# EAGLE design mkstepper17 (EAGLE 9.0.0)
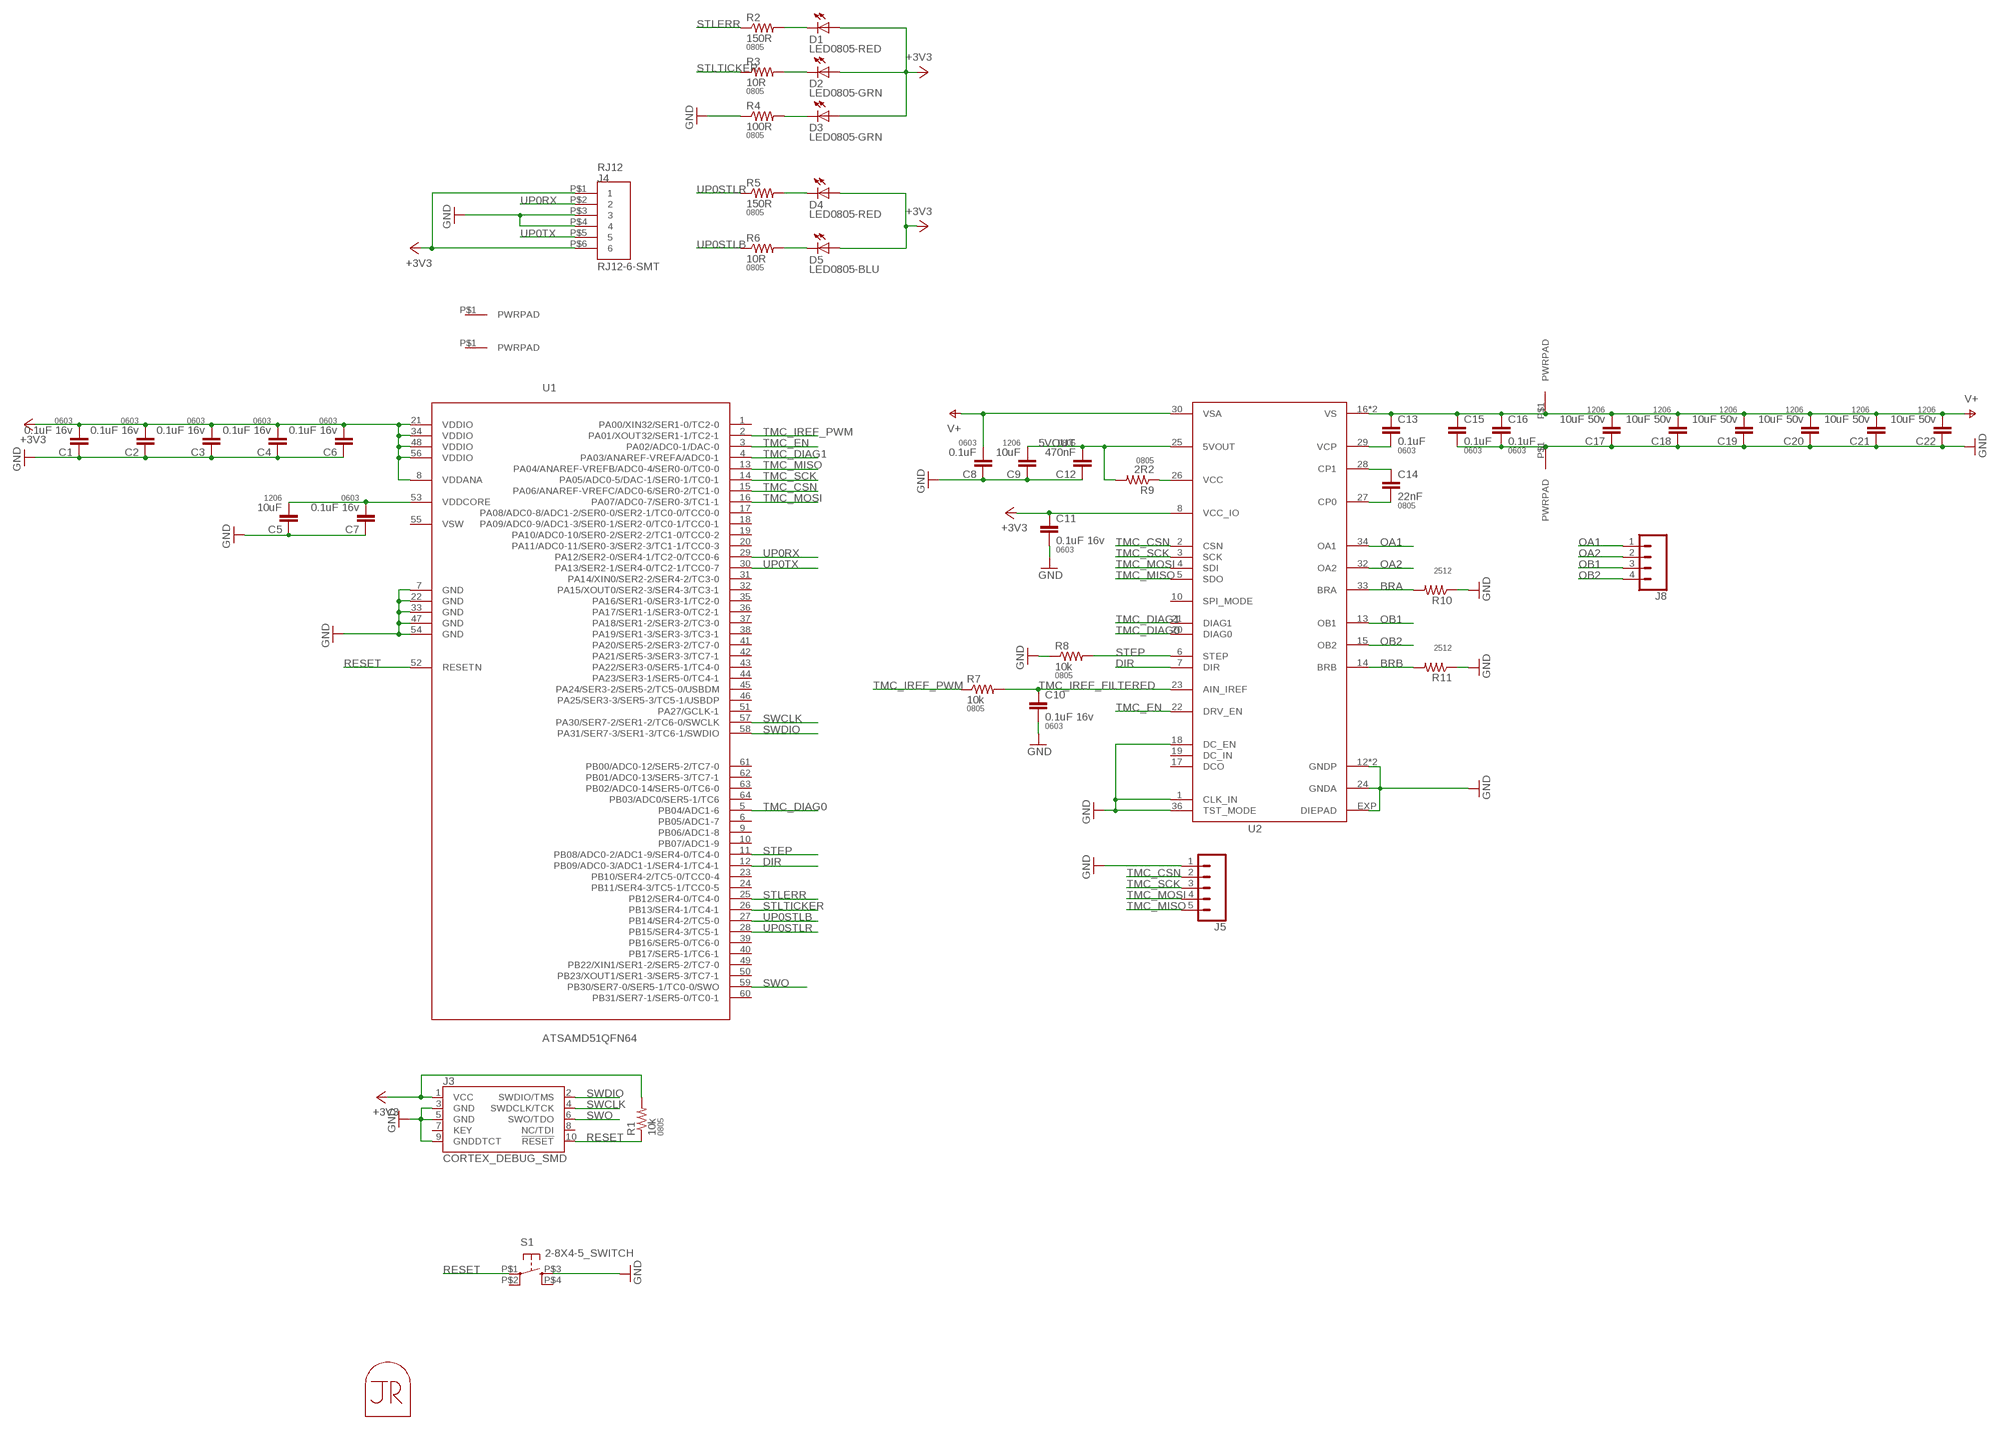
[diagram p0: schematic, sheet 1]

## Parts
C1  0.1uF 16v  CAP0603-CAP  [0603-CAP]
C2  0.1uF 16v  CAP0603-CAP  [0603-CAP]
C3  0.1uF 16v  CAP0603-CAP  [0603-CAP]
C4  0.1uF 16v  CAP0603-CAP  [0603-CAP]
C5  10uF  CAP1206  [1206]
C6  0.1uF 16v  CAP0603-CAP  [0603-CAP]
C7  0.1uF 16v  CAP0603-CAP  [0603-CAP]
C8  0.1uF  CAP0603-CAP  [0603-CAP]
C9  10uF  CAP1206  [1206]
C10  0.1uF 16v  CAP0603-CAP  [0603-CAP]
C11  0.1uF 16v  CAP0603-CAP  [0603-CAP]
C12  470nF  CAP0805  [0805]
C13  0.1uF  CAP0603-CAP  [0603-CAP]
C14  22nF  CAP0805  [0805]
C15  0.1uF  CAP0603-CAP  [0603-CAP]
C16  0.1uF  CAP0603-CAP  [0603-CAP]
C17  10uF 50v  CAP1206  [1206]
C18  10uF 50v  CAP1206  [1206]
C19  10uF 50v  CAP1206  [1206]
C20  10uF 50v  CAP1206  [1206]
C21  10uF 50v  CAP1206  [1206]
C22  10uF 50v  CAP1206  [1206]
D1  LED0805-RED  LED0805  [LED0805]
D2  LED0805-GRN  LED0805  [LED0805]
D3  LED0805-GRN  LED0805  [LED0805]
D4  LED0805-RED  LED0805  [LED0805]
D5  LED0805-BLU  LED0805  [LED0805]
J1  PWRPADM3  [PWRPAD_3-25MM]
J2  PWRPADM3  [PWRPAD_3-25MM]
J3  CORTEX_DEBUG_SMD  [SAMTECH_FTSH-105-01]
J4  RJ12-6-SMT  [RJ12-6-SMT]
J5  CONN_05NO_SILK  [1X05_NO_SILK]
J6  PWRPAD  [PWRPAD_M3-PEM-MOUNT]
J7  PWRPAD  [PWRPAD_M3-PEM-MOUNT]
J8  CONN_04LONGPADS  [1X04_LONGPADS]
MP1  JRTOMBSTONE  [JRTOMBSTONE]
R1  10k  RESISTOR0805-RES  [0805]
R2  150R  RESISTOR0805-RES  [0805]
R3  10R  RESISTOR0805-RES  [0805]
R4  100R  RESISTOR0805-RES  [0805]
R5  150R  RESISTOR0805-RES  [0805]
R6  10R  RESISTOR0805-RES  [0805]
R7  10k  RESISTOR0805-RES  [0805]
R8  10k  RESISTOR0805-RES  [0805]
R9  2R2  RESISTOR0805-RES  [0805]
R10  RESISTOR2512  [R2512]
R11  RESISTOR2512  [R2512]
S1  2-8X4-5_SWITCH  [TACT-SWITCH-KMR6]
U1  ATSAMD51QFN64  [QFN-64-9X9MM]
U2  TMC2130  [QFN36-5X6]

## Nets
5VOUT: C9.2 C12.2 R9.2 U2.25(5VOUT)
+3V3: C1.2 C2.2 C3.2 C4.2 C6.2 C11.1 D1.1(A) D2.1(A) D3.1(A) D4.1(A) D5.1(A) J3.1(VCC) J4.P$1 J4.P$6 R1.2 U1.8(VDDANA) U1.21(VDDIO) U1.34(VDDIO) U1.48(VDDIO) U1.56(VDDIO) U2.8(VCC_IO)
BRA: R10.2 U2.33(BRA)
BRB: R11.2 U2.14(BRB)
DIR: U1.12(PB09/ADC0-3/ADC1-1/SER4-1/TC4-1) U2.7(DIR)
GND: C1.1 C2.1 C3.1 C4.1 C5.1 C6.1 C7.1 C8.1 C9.1 C10.2 C11.2 C12.1 C15.2 C16.2 C17.1 C18.1 C19.1 C20.1 C21.1 C22.1 J3.3(GND) J3.5(GND) J3.9(GNDDTCT) J4.P$3 J4.P$4 J5.1 J7.P$1(PWRPAD) R4.1 R8.1 R10.1 R11.1 S1.P$3(S) U1.7(GND) U1.22(GND) U1.33(GND) U1.47(GND) U1.54(GND) U2.1(CLK_IN) U2.12(GNDP) U2.18(DC_EN) U2.24(GNDA) U2.35(GNDP) U2.36(TST_MODE) U2.EXP(DIEPAD)
N$1: D3.2(C) R4.2
N$5: D2.2(C) R3.2
N$6: D1.2(C) R2.2
N$7: C5.2 C7.2 U1.53(VDDCORE)
N$10: D4.2(C) R5.2
N$11: D5.2(C) R6.2
N$12: C14.2 U2.27(CP0)
N$13: R9.1 U2.26(VCC)
N$14: C14.1 U2.28(CP1)
N$15: C13.2 U2.29(VCP)
OA1: J8.1 U2.34(OA1)
OA2: J8.2 U2.32(OA2)
OB1: J8.3 U2.13(OB1)
OB2: J8.4 U2.15(OB2)
RESET: J3.10(!RESET) R1.1 S1.P$1(P) U1.52(RESETN)
STEP: R8.2 U1.11(PB08/ADC0-2/ADC1-9/SER4-0/TC4-0) U2.6(STEP)
STLERR: R2.1 U1.25(PB12/SER4-0/TC4-0)
STLTICKER: R3.1 U1.26(PB13/SER4-1/TC4-1)
SWCLK: J3.4(SWDCLK/TCK) U1.57(PA30/SER7-2/SER1-2/TC6-0/SWCLK)
SWDIO: J3.2(SWDIO/TMS) U1.58(PA31/SER7-3/SER1-3/TC6-1/SWDIO)
SWO: J3.6(SWO/TDO) U1.59(PB30/SER7-0/SER5-1/TC0-0/SWO)
TMC_CSN: J5.2 U1.15(PA06/ANAREF-VREFC/ADC0-6/SER0-2/TC1-0) U2.2(CSN)
TMC_DIAG0: U1.5(PB04/ADC1-6) U2.20(DIAG0)
TMC_DIAG1: U1.4(PA03/ANAREF-VREFA/ADC0-1) U2.21(DIAG1)
TMC_EN: U1.3(PA02/ADC0-1/DAC-0) U2.22(DRV_EN)
TMC_IREF_FILTERED: C10.1 R7.2 U2.23(AIN_IREF)
TMC_IREF_PWM: R7.1 U1.2(PA01/XOUT32/SER1-1/TC2-1)
TMC_MISO: J5.5 U1.13(PA04/ANAREF-VREFB/ADC0-4/SER0-0/TC0-0) U2.5(SDO)
TMC_MOSI: J5.4 U1.16(PA07/ADC0-7/SER0-3/TC1-1) U2.4(SDI)
TMC_SCK: J5.3 U1.14(PA05/ADC0-5/DAC-1/SER0-1/TC0-1) U2.3(SCK)
UP0RX: J4.P$2 U1.29(PA12/SER2-0/SER4-1/TC2-0/TCC0-6)
UP0STLB: R6.1 U1.27(PB14/SER4-2/TC5-0)
UP0STLR: R5.1 U1.28(PB15/SER4-3/TC5-1)
UP0TX: J4.P$5 U1.30(PA13/SER2-1/SER4-0/TC2-1/TCC0-7)
V+: C8.2 C13.1 C15.1 C16.1 C17.2 C18.2 C19.2 C20.2 C21.2 C22.2 J6.P$1(PWRPAD) U2.16(VS) U2.30(VSA) U2.31(VS)
Unconnected: J1.P$1(PWRPAD) J2.P$1(PWRPAD) J3.7(KEY) J3.8(NC/TDI) S1.P$2(P1) S1.P$4(S1) U1.1(PA00/XIN32/SER1-0/TC2-0) U1.6(PB05/ADC1-7) U1.9(PB06/ADC1-8) U1.10(PB07/ADC1-9) U1.17(PA08/ADC0-8/ADC1-2/SER0-0/SER2-1/TC0-0/TCC0-0) U1.18(PA09/ADC0-9/ADC1-3/SER0-1/SER2-0/TC0-1/TCC0-1) U1.19(PA10/ADC0-10/SER0-2/SER2-2/TC1-0/TCC0-2) U1.20(PA11/ADC0-11/SER0-3/SER2-3/TC1-1/TCC0-3) U1.23(PB10/SER4-2/TC5-0/TCC0-4) U1.24(PB11/SER4-3/TC5-1/TCC0-5) U1.31(PA14/XIN0/SER2-2/SER4-2/TC3-0) U1.32(PA15/XOUT0/SER2-3/SER4-3/TC3-1) U1.35(PA16/SER1-0/SER3-1/TC2-0) U1.36(PA17/SER1-1/SER3-0/TC2-1) U1.37(PA18/SER1-2/SER3-2/TC3-0) U1.38(PA19/SER1-3/SER3-3/TC3-1) U1.39(PB16/SER5-0/TC6-0) U1.40(PB17/SER5-1/TC6-1) U1.41(PA20/SER5-2/SER3-2/TC7-0) U1.42(PA21/SER5-3/SER3-3/TC7-1) U1.43(PA22/SER3-0/SER5-1/TC4-0) U1.44(PA23/SER3-1/SER5-0/TC4-1) U1.45(PA24/SER3-2/SER5-2/TC5-0/USBDM) U1.46(PA25/SER3-3/SER5-3/TC5-1/USBDP) U1.49(PB22/XIN1/SER1-2/SER5-2/TC7-0) U1.50(PB23/XOUT1/SER1-3/SER5-3/TC7-1) U1.51(PA27/GCLK-1) U1.55(VSW) U1.60(PB31/SER7-1/SER5-0/TC0-1) U1.61(PB00/ADC0-12/SER5-2/TC7-0) U1.62(PB01/ADC0-13/SER5-3/TC7-1) U1.63(PB02/ADC0-14/SER5-0/TC6-0) U1.64(PB03/ADC0/SER5-1/TC6) U2.10(SPI_MODE) U2.17(DCO) U2.19(DC_IN)

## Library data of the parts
C1-C4 C6-C8 C10 C11 C13 C15 C16 = borkedlabs-passives:CAP: Capacitor; PACKAGE: 0603
C5 C9 C17-C22 = borkedlabs-passives:CAP: Capacitor; PACKAGE: 1206
C12 C14 = borkedlabs-passives:CAP: Capacitor; PACKAGE: 0805
D1-D5 = lights:LED: LED
J1 J2 J6 J7 = power:PWRPAD
J3 = SparkFun-Connectors:CORTEX_DEBUG: Cortex Debug Connector - 10 pin Supports JTAG debug, Serial Wire debug, and Serial Wire Viewer. PTH and SMD connector options available. General Connector Information Products: PTH Connector -via Digi-Key SparkFun PSoc SparkFun T
J4 = connector:RJ12-6-SMT
J5 = SparkFun-Connectors:CONN_05: Multi connection point. Often used as Generic Header-pin footprint for 0.1 inch spaced/style header connections On any of the 0.1 inch spaced packages, you can populate with these: Break Away Headers - Straight (PRT-00116) Break Away Male Headers - Right Angle (PRT-00553) Female Headers (PRT-00115)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
J8 = SparkFun-Connectors:CONN_04: Multi connection point. Often used as Generic Header-pin footprint for 0.1 inch spaced/style header connections On any of the 0.1 inch spaced packages, you can populate with these: Break Away Headers - Straight (PRT-00116) Break Away Male Headers - Right Angle (PRT-00553) Female Headers (PRT-00115)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; PROD_ID: CONN-09696
MP1 = connector:JRTOMBSTONE
R1-R9 = borkedlabs-passives:RESISTOR: Resistor; PACKAGE: 0805
R10 R11 = borkedlabs-passives:RESISTOR: Resistor; PACKAGE: 2512
S1 = fab:2-8X4-5_SWITCH
U1 = atsam:ATSAMD51
U2 = power:TMC2130

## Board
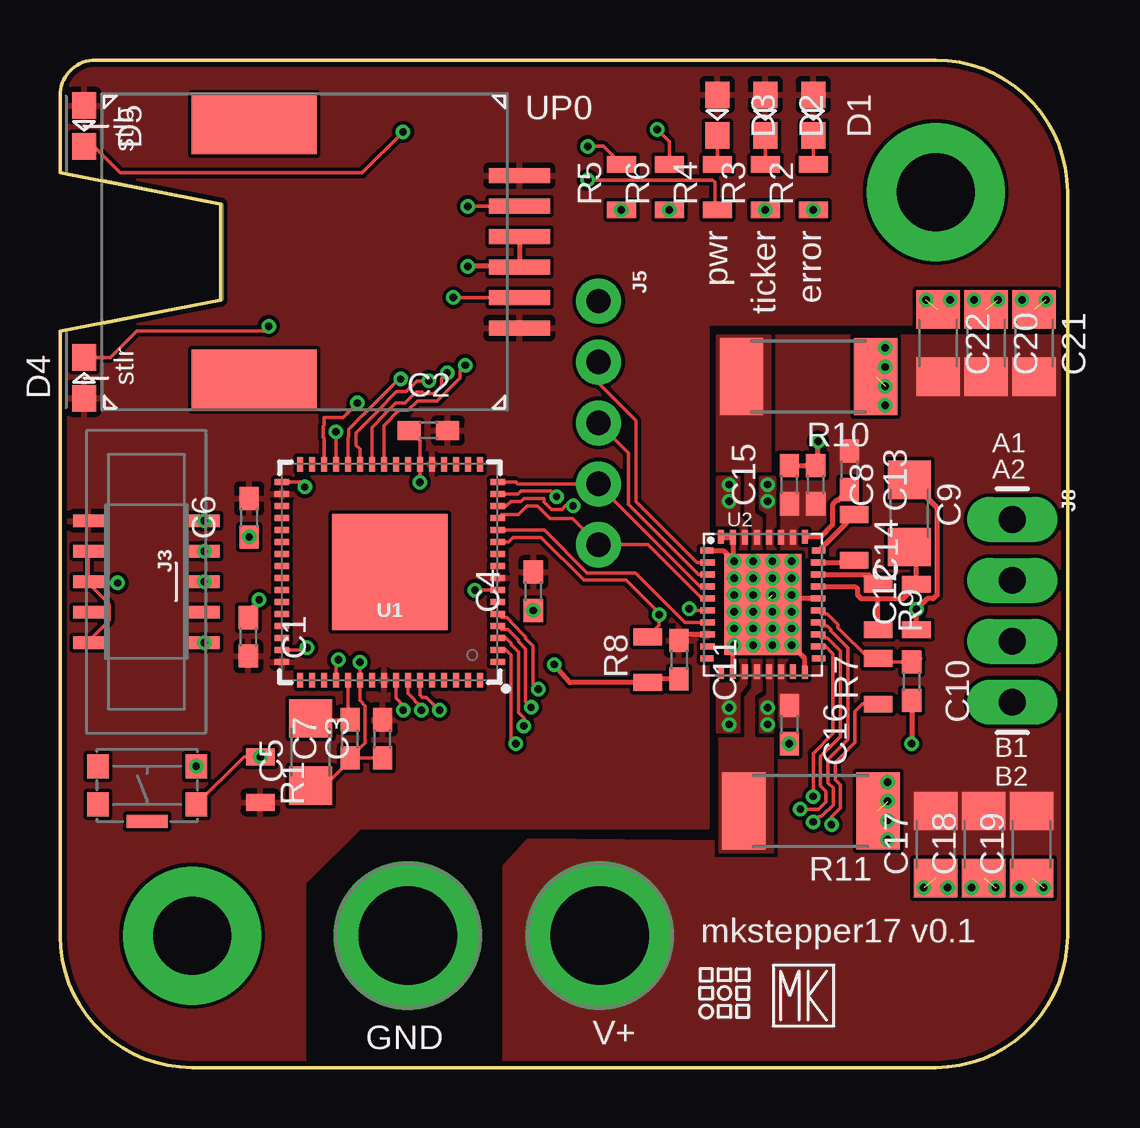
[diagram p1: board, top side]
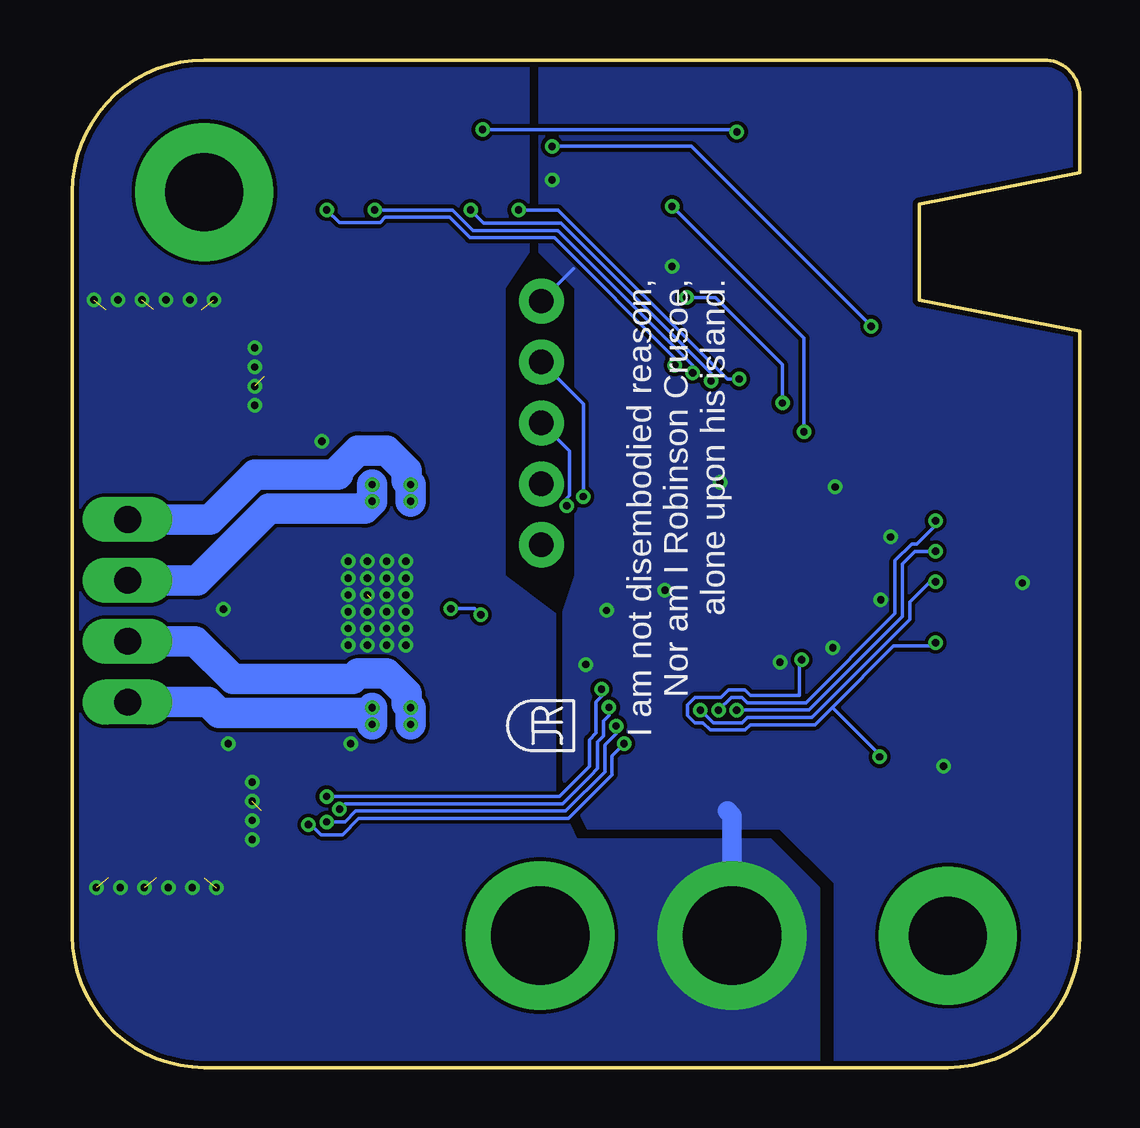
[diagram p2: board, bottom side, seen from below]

Size 42 x 42 mm. Coordinates in mm from the lower left corner, seen from the top.
Outline: 5.5,0 36.5,0 arc90 42,5.5 42,36.5 arc90 36.5,42 1.5,42 arc90 0,40.5 0,37.3 6.7,36 6.7,32 0,30.7 0,5.5 arc90 5.5,0
Copper layers (1*16): Top 0.035mm / dielectric 1.5mm / Bottom 0.035mm
Design rules "default *": minimum track width 6mil, minimum drill 0.3mm, track to track 6mil, track to pad 6mil, pad to pad 6mil, via to via 6mil, smd to smd 6mil, copper to edge 8mil, drill to drill 8mil, minimum pad ring 6mil, minimum via ring 6mil, stop-mask expansion 4mil, vias tented up to drill 27mil, thermal gap 9mil

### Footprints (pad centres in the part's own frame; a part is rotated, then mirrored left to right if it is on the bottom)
0603-CAP = smd 0.96 x 0.8: 1 -0.8,0; 2 0.8,0
1206 = smd 1.6 x 1.8: 1 -1.4,0; 2 1.4,0
0805 = smd 0.7 x 1.2: 1 -0.95,0; 2 0.95,0
LED0805 = smd 1.1 x 1: 1 -0.85,0; 2 0.85,0
PWRPAD_3-25MM = drill 3.25 pad 5.75: P$1 0,0
SAMTECH_FTSH-105-01 = smd 0.508 x 1.27: 1 -2.54,-2.413; 2 -2.54,2.413; 3 -1.27,-2.413; 4 -1.27,2.413; 5 0,-2.413; 6 0,2.413; 7 1.27,-2.413; 8 1.27,2.413; 9 2.54,-2.413; 10 2.54,2.413
RJ12-6-SMT = smd 0.635 x 2.54: P$1 -3.175,17.399; P$2 -1.905,17.399; P$3 -0.635,17.399; P$4 0.635,17.399; P$5 1.905,17.399; P$6 3.175,17.399 | smd 2.54 x 5.207: P$7 -5.334,6.35; P$8 5.334,6.35
1X05_NO_SILK = drill 1.016 pad 1.88: 1 0,0; 2 2.54,0; 3 5.08,0; 4 7.62,0; 5 10.16,0
PWRPAD_M3-PEM-MOUNT = drill 4.1 pad 6.2: P$1 0,0
1X04_LONGPADS = drill 1.118 pad 1.88 long: 1 0,0; 2 2.54,0; 3 5.08,0; 4 7.62,0
R2512 = smd 1.8 x 3.2: 1 -2.8,0; 2 2.8,0
TACT-SWITCH-KMR6 = smd 0.9 x 1: P$1 -2.05,0.8; P$2 2.05,0.8; P$3 -2.05,-0.8; P$4 2.05,-0.8 | smd 1.7 x 0.55: P$5 0,1.5
QFN-64-9X9MM = smd 0.6 x 0.25: 1 -4.5,3.75; 2 -4.5,3.25; 3 -4.5,2.75; 4 -4.5,2.25; 5 -4.5,1.75; 6 -4.5,1.25; 7 -4.5,0.75; 8 -4.5,0.25; 9 -4.5,-0.25; 10 -4.5,-0.75; 11 -4.5,-1.25; 12 -4.5,-1.75; 13 -4.5,-2.25; 14 -4.5,-2.75; 15 -4.5,-3.25; 16 -4.5,-3.75; 33 4.5,-3.75; 34 4.5,-3.25; 35 4.5,-2.75; 36 4.5,-2.25; 37 4.5,-1.75; 38 4.5,-1.25; 39 4.5,-0.75; 40 4.5,-0.25; 41 4.5,0.25; 42 4.5,0.75; 43 4.5,1.25; 44 4.5,1.75; 45 4.5,2.25; 46 4.5,2.75; 47 4.5,3.25; 48 4.5,3.75 | smd 0.25 x 0.6: 17 -3.75,-4.5; 18 -3.25,-4.5; 19 -2.75,-4.5; 20 -2.25,-4.5; 21 -1.75,-4.5; 22 -1.25,-4.5; 23 -0.75,-4.5; 24 -0.25,-4.5; 25 0.25,-4.5; 26 0.75,-4.5; 27 1.25,-4.5; 28 1.75,-4.5; 29 2.25,-4.5; 30 2.75,-4.5; 31 3.25,-4.5; 32 3.75,-4.5; 49 3.75,4.5; 50 3.25,4.5; 51 2.75,4.5; 52 2.25,4.5; 53 1.75,4.5; 54 1.25,4.5; 55 0.75,4.5; 56 0.25,4.5; 57 -0.25,4.5; 58 -0.75,4.5; 59 -1.25,4.5; 60 -1.75,4.5; 61 -2.25,4.5; 62 -2.75,4.5; 63 -3.25,4.5; 64 -3.75,4.5 | smd 4.826 x 4.826: P$1 0,0
QFN36-5X6 = smd 0.55 x 0.25: 1 -2.325,1.75; 10 -2.325,-2.75; 19 2.325,-2.75; 28 2.325,1.75 | smd 0.6 x 0.25: 2 -2.3,1.25; 3 -2.3,0.75; 4 -2.3,0.25; 5 -2.3,-0.25; 6 -2.3,-0.75; 7 -2.3,-1.25; 8 -2.3,-1.75; 9 -2.3,-2.25; 20 2.3,-2.25; 21 2.3,-1.75; 22 2.3,-1.25; 23 2.3,-0.75; 24 2.3,-0.25; 25 2.3,0.25; 26 2.3,0.75; 27 2.3,1.25 | smd 0.25 x 0.55: 11 -1.75,-3.325; 18 1.75,-3.325; 29 1.75,2.325; 36 -1.75,2.325 | smd 0.25 x 0.6: 12 -1.25,-3.3; 13 -0.75,-3.3; 14 -0.25,-3.3; 15 0.25,-3.3; 16 0.75,-3.3; 17 1.25,-3.3; 30 1.25,2.3; 31 0.75,2.3; 32 0.25,2.3; 33 -0.25,2.3; 34 -0.75,2.3; 35 -1.25,2.3 | smd 3.2 x 4.2: EXP 0,-0.5

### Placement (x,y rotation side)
C1  7.85,17.95 270 top
C2  15.36,26.55 0 top
C3  13.45,13.7 90 top
C4  19.73,19.85 90 top
C5  10.45,13.15 90 top
C6  7.89,22.92 90 top
C7  12.1,13.7 90 top
C8  31.5,24.3 270 top
C9  35.4,23.1 270 top
C10  35.5,16.1 270 top
C11  25.8,17 270 top
C12  35.7,19.2 90 top
C13  32.9,24.9 270 top
C14  33.1,22.1 270 top
C15  30.4,24.3 90 top
C16  30.4,14.3 270 top
C17  36.5,9.3 90 top
C18  38.5,9.3 90 top
C19  40.5,9.3 90 top
C20  38.6,30.2 270 top
C21  40.6,30.2 270 top
C22  36.6,30.2 270 top
D1  31.4,39.7 270 top
D2  29.4,39.7 270 top
D3  27.4,39.7 270 top
D4  1,28.75 90 top
D5  1,39.25 270 top
J1  36.5,36.5 0 top
J2  5.5,5.5 0 top
J3  3.6,20.25 270 top
J4  1.75,34 270 top
J5  22.45,31.95 270 top
J6  22.5,5.5 0 top
J7  14.5,5.5 0 top
J8  39.7,22.85 270 top
MP1  22.1,14.3 90 bottom
R1  8.35,12 270 top
R2  31.4,36.7 90 top
R3  29.4,36.7 90 top
R4  27.4,36.7 90 top
R5  23.4,36.7 90 top
R6  25.4,36.7 90 top
R7  34.1,16.1 90 top
R8  24.5,17 90 top
R9  34.1,19.2 270 top
R10  31.2,28.8 180 top
R11  31.3,10.7 180 top
S1  3.63,11.76 180 top
U1  13.75,20.65 180 top
U2  29.3,19.8 0 top
U$5  [CBA-SILK-LOGO]  27.7,3.1 90 top
U$9  [MK-LOGO-SILK]  31,3 0 top

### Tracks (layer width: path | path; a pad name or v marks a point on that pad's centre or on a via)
5VOUT
  Top 0.203: C12.2 35.8,20.35 | C12.2 35.7,20.1 35.15,19.55 34.1,19.55 | C12.2 35.7,21.4 C9.2 | U2.25 33.15,20.05 33.25,19.95 33.25,19.7 33.4,19.55 34.1,19.55 | R9.2 34.1,19.55
+3V3
  Top 0.203: U2.8 26.05,18.05 C11.1
  pour Top: 45,31 27,31 27,10 12.5,10 10.2,7.7 10.2,-1 -1,-1 -1,44 45,44
BRA
  pour Top (rank 4, no thermals): 27.4,21.4 27.4,30.5 29.6,30.5 29.6,21.4
BRB
  pour Top (rank 4, no thermals): 27.5,9 27.5,18.1 29.7,18.1 29.7,9
DIR
  Top 0.152: U1.12 20.19,22.4 21.97,20.62 23.98,20.62 26.05,18.55 U2.7
GND  (via drill 0.3)  (9 unrouted)
  Top 0.152: 28.05,21.05 v28.1,21.1 | 28.05,18.05 U2.EXP | U1.7 v17.3,19.9 | v15,24.4 U1.22 15,26.11 C2.1 | U1.33 10,24.4 v10.2,24.2 | U1.47 10.2,17.4 v10.3,17.5 | v12.5,16.9 U1.54 12.5,15.3 12.73,15.07 12.73,13.53 12.15,12.95 | 12.15,12.95 C7.1 | C3.1 12.2,12.9 | 12.2,12.9 12.15,12.95 | C5.1 11.05,11.75 12.2,12.9 | C1.1 7.85,19.05 v8.3,19.5 | J3.3 J3.5 | J3.5 1.19,20.19 2.05,19.33 2.05,18.63 1.19,17.77 J3.9 | J3.5 1.24,20.2 v2.4,20.2 | R4.1 27.3,35.85 27.3,36.9 27.2,37 v22,37
  Top 0.203: U2.24 29.55,19.55 U2.EXP | C9.1 36.55,23.35 36.55,19.7 36.41,19.55 36.15,19.55 v35.7,19.1 C12.1 | C10.2 v35.5,13.5 | C15.2 C8.1 31.6,25.2 v31.6,26.1 | C11.2 24.65,16.2 R8.1 21.25,16.05 v20.6,16.8 | J4.P$3 J4.P$4 19.11,33.4 v17,33.4 | U2.12 28.05,17.55 v28.1,17.6 | 28.05,21.15 U2.35 27.57,22.1 U2.36 | 28.05,21.15 v28.1,21.1 | U2.1 27.65,21.55 28.05,21.15 | U2.18 31.05,17.05 v30.5,17.6
  Bottom 0.152: J5.1 21.1,33.3
  Bottom 0.813: J7.P$1 14.5,10.5 14.7,10.7
  other vias: 30.5,20.4 29.7,20.4 28.9,20.4 28.1,20.4 28.9,18.3 28.9,19 28.1,18.3 28.1,19 29.7,19 29.7,18.3 30.5,18.3 30.5,19 28.1,19.7 28.9,19.7 29.7,19.7 30.5,19.7 30.4,13.5 19.73,19.05 7.89,22.12 5.68,12.56 28.9,17.6 29.7,17.6 30.5,21.1 29.7,21.1 28.9,21.1 34.4,30 34.4,29.2 34.4,27.6 34.4,28.4 36.1,32 37.1,32 38.1,32 39.1,32 40.1,32 41.1,32 36,7.5 37,7.5 38,7.5 39,7.5 40,7.5 41,7.5 34.5,9.5 34.5,11.9 34.5,10.3 34.5,11.1
  pour Bottom: 23,43.5 23,34 24,32.5 24,20.5 21.9,18.9 21.9,11.4 21,9.5 12.9,9.5 10.9,7.5 10.9,-2.5 44.5,-2.5 44.5,43.5
  pour Bottom: 22.5,44.5 22.5,34 21,32.5 21,20.5 21.5,19 21.5,12 20.5,10 12.5,10 10.2,7.7 10.2,-1 -1.5,-1 -1.5,44.5
N$1
  Top 0.152: D3.2 R4.2
N$5
  Top 0.152: D2.2 R3.2
N$6
  Top 0.152: D1.2 R2.2
N$7
  Top 0.152: U1.53 12,14.7 C7.2 10.7,14.5 C5.2
N$10  (via drill 0.3)
  Top 0.152: R5.2 22.65,38.4 v22,38.4 | v8.7,30.9 8.5,30.7 3.2,30.7 2.1,29.6 D4.2
  Bottom 0.152: v22,38.4 16.2,38.4 v8.7,30.9
N$11  (via drill 0.3)
  Top 0.152: D5.2 1.4,38.4 2.5,37.3 12.6,37.3 v14.3,39 | v24.9,39.1 25.4,38.6 R6.2
  Bottom 0.152: v14.3,39 14.4,39.1 v24.9,39.1
N$12
  Top 0.203: U2.27 32.7,21.05 C14.2
N$13
  Top 0.203: R9.1 33.7,20.55 33.51,20.55 32.09,20.55 U2.26
N$14
  Top 0.203: U2.28 32.8,22.73 C14.1
N$15
  Top 0.203: C13.2 32.45,23.65 32.4,23.65 32.2,23.46 32.2,22.63 31.7,22.12 U2.29
OA1  (via drill 0.3)
  Bottom 1.27: J8.1 36.26,22.85 34.39,24.72 30.92,24.72 30.92,24.89 30.09,25.72 28.91,25.72 28.08,24.89 28.08,24.48 v27.9,24.3 v27.9,23.6
  pour Top (no thermals): 28.3,21.4 28.3,22.6 27.4,22.6 27.4,24.6 28.3,24.6 28.3,23 28.6,22.6 28.6,21.4
OA2  (via drill 0.3)
  Bottom 1.27: v29.5,24.3 v29.5,23.6 29.8,23.3 33.8,23.3 36.8,20.3 39.49,20.3 J8.2
  pour Top (no thermals): 29.5,21.4 29.5,23.1 29.2,23.3 29.2,24.6 29.8,24.6 29.8,21.4
OB1  (via drill 0.3)
  Bottom 1.27: v27.9,14.3 v27.9,15 28.08,15.18 28.08,15.59 28.91,16.42 30.09,16.42 30.31,16.2 35.3,16.2 36.87,17.77 J8.3
  pour Top (no thermals): 28.3,17.2 28.3,16 27.4,16 27.4,14 28.3,14 28.3,15.6 28.6,16 28.6,17.2
OB2  (via drill 0.3)
  Bottom 1.27: v29.5,14.3 v29.5,15 29.72,14.78 35.89,14.78 36.34,15.23 J8.4
  pour Top (no thermals): 29.5,17.2 29.5,15.5 29.2,15.3 29.2,14 29.7,14 29.7,17.2
RESET  (via drill 0.3)
  Top 0.152: U1.52 11.5,16.9 v11.6,17 | S1.P$1 7.67,12.95 R1.1
  Bottom 0.152: v11.6,17 11.7,16.9 11.7,15.51 13.73,15.51 13.96,15.74 14.66,15.74 14.96,15.43 16.04,15.43 16.35,15.12 16.35,14.68 16.04,14.37 15.71,14.37 15.41,14.06 13.96,14.06 13.73,14.29 11.05,14.29 10.32,15.02 | 10.32,15.02 7.77,17.57 6.15,17.57 J3.10 | R1.1 8.35,13.05 10.32,15.02
  other vias: 6.01,17.71 8.35,12.95
STEP  (via drill 0.3)
  Top 0.152: U2.6 26.3,19.05 v26.23,19.13 | R8.2 24.98,18.43 v24.98,18.88 24.98,18.94 23.6,20.32 21.84,20.32 20.06,22.09 18.89,22.09 18.7,21.9 U1.11
  Bottom 0.152: v26.23,19.13 25.23,19.13 v24.98,18.88
STLERR  (via drill 0.3)
  Top 0.152: v16.89,29.28 16.67,29.06 16.67,28.74 15.72,27.79 14.9,27.79 14.51,27.4 14.14,27.4 13.5,26.76 U1.25
  Bottom 0.152: R2.1 30.87,35.22 29.18,35.22 28.95,35.45 26.28,35.45 25.42,34.59 21.9,34.59 16.81,29.5 16.79,29.5 16.65,29.35 16.82,29.35 v16.89,29.28
  other vias: 31.4,35.75
STLTICKER  (via drill 0.3)
  Top 0.152: v16.14,28.96 15.91,28.72 15.91,28.41 15.59,28.09 15.16,28.09 15.09,28.16 14.84,28.16 14.39,27.7 14,27.7 13.54,27.25 13.54,27.23 13,26.69 U1.26
  Bottom 0.152: v16.14,28.96 16.14,29.28 21.76,34.9 25.3,34.9 26.15,35.75 R3.1
  other vias: 29.4,35.75
SWCLK  (via drill 0.3)
  Top 0.152: U1.57 14,15.4 14.3,15.09 v14.3,14.9
  Bottom 0.152: v14.3,14.9 11.3,14.9 7.4,18.8 7.4,21 6.88,21.52 J3.4
  other vias: 6.01,21.52
SWDIO  (via drill 0.3)
  Top 0.152: U1.58 14.5,15.6 15.06,15.04 v15.06,14.9
  Bottom 0.152: v15.06,14.9 14.53,15.43 14.09,15.43 13.86,15.2 11.43,15.2 7.71,18.93 7.71,21.13 7.01,21.82 6.8,21.82 6.01,22.61 J3.2
  other vias: 6.01,22.79
SWO  (via drill 0.3)
  Top 0.152: U1.59 15,15.53 15.1,15.43 15.28,15.43 15.59,15.12 15.59,14.94 15.63,14.9 v15.82,14.9
  Bottom 0.152: v15.82,14.9 v15.81,14.9 15.28,14.37 14.09,14.37 13.86,14.59 11.17,14.59 7.1,18.67 7.1,19.4 6.24,20.25 J3.6
  other vias: 6.01,20.25
TMC_CSN  (via drill 0.3)
  Top 0.152: U2.2 26.54,21.05 24,23.59 24,26.97 22.45,28.52 J5.2 | U1.15 19.1,23.9 19.23,24.02 20.47,24.02 v20.7,23.8
  Bottom 0.152: v20.7,23.8 20.7,27.66 J5.2
TMC_DIAG0  (via drill 0.3)
  Top 0.152: U2.20 31.92,17.55 32.23,17.25 32.23,13.93 31.4,13.1 v31.4,11.3 | v19.94,15.77 19.71,16 19.71,17.58 19.41,17.88 19.41,17.95 18.78,18.58 18.78,18.62 18.64,18.75 18.4,18.75 U1.5
  Bottom 0.152: v31.4,11.3 21.7,11.3 20.45,12.55 20.45,13.66 20.17,13.94 20.17,15.23 19.94,15.46 v19.94,15.77
TMC_DIAG1  (via drill 0.3)
  Top 0.152: U2.21 31.75,17.9 32,17.9 32.53,17.37 32.53,13.8 31.7,12.97 31.7,11.75 31.93,11.52 31.93,11.08 31.62,10.77 v30.86,10.77 | U1.4 18.4,18.25 18.68,18.25 19.11,17.83 19.11,17.76 19.41,17.45 19.41,15.24 v19.64,15.02
  Bottom 0.152: v30.86,10.77 30.63,10.99 21.57,10.99 20.28,12.28 20.23,12.33 20.11,12.46 20.11,13.57 19.87,13.82 19.87,14.45 19.64,14.69 v19.64,15.02
TMC_EN  (via drill 0.3)
  Top 0.152: U2.22 31.75,18.4 31.99,18.4 32.13,18.27 32.13,18.2 32.84,17.5 32.84,13.67 32.01,12.85 32.01,11.87 32.24,11.65 32.24,10.95 31.75,10.46 31.63,10.46 v31.4,10.24 | v19.34,14.23 19.34,14.57 19.11,14.8 19.11,17.33 18.8,17.63 18.8,17.7 18.6,17.9 U1.3
  Bottom 0.152: v31.4,10.24 30.64,10.24 30.19,10.69 21.45,10.69 19.8,12.33 19.8,13.45 19.34,13.92 v19.34,14.23
TMC_IREF_FILTERED
  Top 0.152: U2.23 31.75,18.9 31.99,18.9 32.43,18.46 32.43,18.33 33.71,17.05 R7.2 34.25,16.9 C10.1
  Top 0.203: 35.85,17.05 C10.1
TMC_IREF_PWM  (via drill 0.3)
  Top 0.152: R7.1 33.45,15.15 33.14,14.84 33.14,13.55 32.31,12.72 32.31,12 32.54,11.77 32.54,10.83 32.16,10.44 v32.16,10.12 | U1.2 18.6,17.4 18.8,17.2 18.8,13.7 v19,13.5
  Bottom 0.152: v32.16,10.12 32.04,10.12 31.62,9.71 30.74,9.71 30.06,10.39 21.32,10.39 19.5,12.21 19.5,13 v19,13.5
TMC_MISO
  Top 0.152: U2.5 26.75,19.55 24.5,21.8 J5.5 | J5.5 | U1.13 18.4,23.05 19.11,23.05 19.48,23.42 19.9,23.42 20.43,22.89 21.37,22.89 J5.5
TMC_MOSI
  Top 0.152: U2.4 26.68,20.05 22.45,24.28 J5.4 19.07,24.33 19,24.4 U1.16
TMC_SCK  (via drill 0.3)
  Top 0.152: U2.3 26.61,20.55 23.7,23.46 23.7,25.62 J5.3 | U1.14 18.6,23.4 18.8,23.59 19.23,23.59 19.35,23.72 20.17,23.72 20.17,23.58 20.48,23.27 20.92,23.27 21.07,23.42 v21.39,23.42
  Bottom 0.152: v21.39,23.42 21.39,23.74 21.28,23.85 21.28,25.7 J5.3
UP0RX  (via drill 0.3)
  Top 0.152: v17,35.9 v17,35.91 J4.P$2 | U1.29 v11.5,26.5
  Bottom 0.152: v11.5,26.5 11.5,30.4 v17,35.9
UP0STLB  (via drill 0.3)
  Top 0.152: v15.38,28.62 14.88,28.62 14.42,28.17 14.03,28.17 13.24,27.37 13.24,27.35 12.34,26.45 12.34,25.94 12.5,25.77 U1.27
  Bottom 0.152: R6.1 24.85,35.2 21.63,35.2 15.38,28.94 v15.38,28.62
  other vias: 25.4,35.75
UP0STLR  (via drill 0.3)
  Top 0.152: U1.28 12,26.25 12.03,26.28 12.03,26.6 12.6,27.17 12.62,27.17 12.93,27.48 12.93,27.5 14.13,28.7 v14.2,28.7
  Bottom 0.152: v14.2,28.7 14.7,28.7 21.75,35.75 R5.1
  other vias: 23.4,35.75
UP0TX  (via drill 0.3)
  Top 0.152: J4.P$5 v16.41,32.09 v16.4,32.1 | v12.4,27.7 11.8,27.1 11,27.1 11,26.75 10.97,26.72 10.97,26.28 11,26.25 U1.30
  Bottom 0.152: v16.4,32.1 15.2,32.1 12.4,29.3 v12.4,27.7
V+
  pour Top (rank 5, no thermals): 44.5,30.5 27.5,30.5 27.6,9.4 19.5,9.5 18.5,8.4 18.5,-0.6 19.6,-1 44.5,-1

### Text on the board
tPlace: UP0 | pwr | ticker | error | A1 | A2 | B1 | B2 | mkstepper17 v0.1 | GND | V+
bPlace: I am not disembodied reason, / Nor am I Robinson Crusoe, / alone upon his island.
